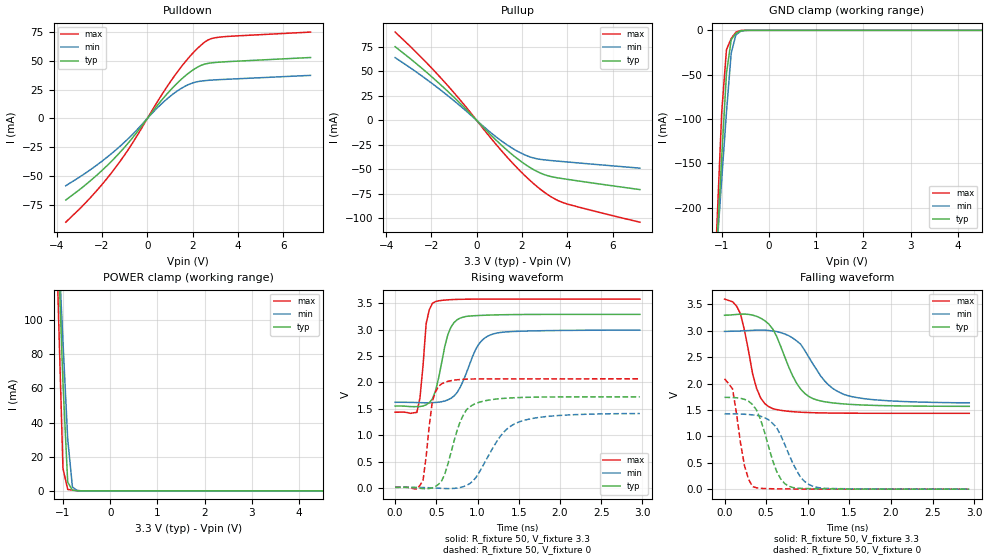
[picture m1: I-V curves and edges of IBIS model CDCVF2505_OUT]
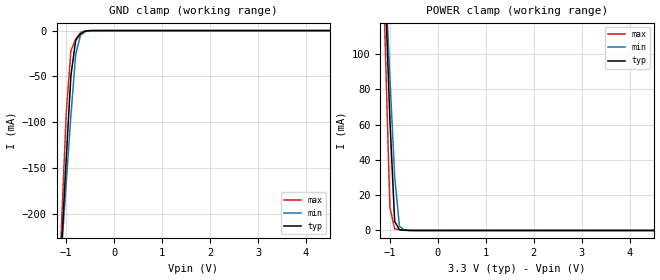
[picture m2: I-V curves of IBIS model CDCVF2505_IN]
|   TEXAS INSTRUMENTS INCORPORATED
|   CLOCK DISTRIBUTION CIRCUITS
|   IBIS Model of CDCVF2505
|   3.3-V High Performance PLL Clock Buffer
|   8-pin (PW(R), D(R)) Package
[IBIS Ver]   3.2
[File Name]   vf2505_2.ibs
[File Rev]   0.9
[Date]   Sept 6th 2005
[Source]   File originated at Texas Instruments, Inc.
[Notes]   The following is an IBIS list for the CDCVF2310.
|   - All test data contained in this file are derived from
|   hspice(tm) simulations.
|   - File created by HPA-Product Engineering.
|   01: model based on VF2310 simulation data. Tr seems to be about
|   200ps too fast compared to device characterization data.
|   0.8: Model correlated finally with updated package parasitics
|   to real silicon measurements.
|   0.9: Switched the definition of CLK_OUT pin - uses the same output model as the outputs 1Y0...1Y3.
|   But this pin is internally connected to "FBIN". C_comp therefore is different. In order to separately
|   add model data for this pin, also Hspice simulations would be needed. This pin normally is not used
|   in application to drive system loads. It acts mainly for phase adjustments to get the correct phase
|   between CLK and output buffers. But this effect is not modeled in IBIS.
|   If a customer needs this pin to drive system load, one may consider to increase C_comp by 2.4pF.
[Disclaimer] Property of Texas Instruments Incorporated.  Unauthorized
   reproduction and/or distribution is strictly prohibited.
   This product is protected under copyright law.
   Created 2004, (C) Copyright 2004, Texas Instruments Inc.,
   All Rights Reserved
   UNLESS THERE IS A SIGNED, WRITTEN AGREEMENT TO THE
   CONTRARY, TEXAS INSTRUMENTS ("TI") IS PROVIDING THE IBIS
   MODELS "AS IS" AND WITHOUT ANY WARRANTY, EXPRESSED OR
   IMPLIED.  TI assumes no liability for:
   1) the accuracy of the IBIS models provided to your
   company;
   2) the proper functioning of these IBIS models in your
   design or for any resulting applications; or
   3) infringement of patents, copyrights or intellectual
   property rights resulting from your use of these IBIS
   models.
   TI provides IBIS Models as a service to our customers.
   You and your company shall not distribute, sell or give
   these models to anyone else without prior written
   permission from TI.
   TI reserves the right to make changes to our products or
   to discontinue any semiconductor product or service
   without notice, and advises our customers to obtain the
   latest version of relevant information to verify, before
   placing orders, that the information being relied on is
   current.
   Please be aware that your receipt and use of the IBIS
   information provided shall serve as acceptance of these
   terms and conditions.  If you do not accept these terms,
   you should return or destroy the IBIS models and any
   other accompanying information immediately.
|   Model CDCVF2505PW(R)
[Component]   CDCVF2505PW   | (High_Performance_Clock_Buffer)
[Manufacturer]  Texas Instruments, Inc.
[Package]
|   typ   min   max
R_pkg   0.097ohm   0.067ohm   0.115ohm
L_pkg   3.349nH   2.836nH   3.571nH
C_pkg   0.308pF   0.263pF   0.371pF
[Pin]   signal_name   model_name   R_pin   L_pin   C_pin
  1   CLKIN   CDCVF2505_IN   0.099Ohm   3.541nH   0.343pF
  2   1Y1   CDCVF2505_OUT   0.104Ohm   3.297nH   0.263pF
  3   1Y0   CDCVF2505_OUT   0.109Ohm   3.365nH   0.272pF
  4   GND   GND   0.081Ohm   3.275nH   0.371pF
  5   1Y2   CDCVF2505_OUT   0.098Ohm   3.479nH   0.340pF
  6   VDD   POWER   0.067Ohm   2.836nH   0.319pF
  7   1Y3   CDCVF2505_OUT   0.115Ohm   3.430nH   0.275pF
| 8   CLKOUT   CDCVF2505_CLKOUT   0.102Ohm   3.571nH   0.284pF
|   Model CDCVF2505D(R)
[Component]   CDCVF2505D   | (High_Performance_Clock_Buffer)
[Manufacturer]  Texas Instruments, Inc.
[Package]
|   typ   min   max
R_pkg   0.087ohm   0.041ohm   0.113ohm
L_pkg   1.932nH   1.186nH   2.417nH
C_pkg   0.410pF   0.344pF   0.540pF
[Pin]   signal_name   model_name   R_pin   L_pin   C_pin
  1   CLKIN   CDCVF2505_IN   0.110Ohm   2.376nH   0.429pF
  2   1Y1   CDCVF2505_OUT   0.088Ohm   1.771nH   0.344pF
  3   1Y0   CDCVF2505_OUT   0.086Ohm   1.750nH   0.346pF
  4   GND   GND   0.060Ohm   1.756nH   0.540pF
  5   1Y2   CDCVF2505_OUT   0.111Ohm   2.400nH   0.429pF
  6   VDD   POWER   0.041Ohm   1.186nH   0.416pF
  7   1Y3   CDCVF2505_OUT   0.090Ohm   1.797nH   0.345pF
  8   CLKOUT   CDCVF2505_OUT   0.113Ohm   2.417nH   0.432pF
| Models and submodels in the file (2): CDCVF2505_OUT (3-state), CDCVF2505_IN (Input)
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|   Model CDCVF2505_OUT
[Model]   CDCVF2505_OUT
Model_type   3-state
Polarity   Non-Inverting
Enable   Active-High
Vmeas = 1.65V   |Vref for timing measurements.
Cref = 25pF   |load capacitance for timing spec.
Rref = 500   |500 Ohm to GND.
Vref = 0   |Timing specification test load voltage, GND
| variable   typ   min   max
C_comp   2.5pF   NA   NA
[Model Spec]
|  subparameter   typ   min   max
Vmeas   1.65V   1.5V   1.80V
[Temperature Range]   40   85   -40
[Voltage range]   3.3   3.0   3.6
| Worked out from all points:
|   slope of the pulldown table from 0 to 0.495 V, typ, clamps not added: 39.3 ohm
|   slope of the pullup table from 0 to 0.495 V, typ, clamps not added: 41.4 ohm
|   GND clamp passes 1 mA (typ) near -0.61 V on its own axis
|   POWER clamp passes 1 mA (typ) near -0.81 V on its own axis
|   rising waveform, R_fixture 50, V_fixture 3.3: 20-80 % time 151ps typ, 227ps min, 70.9ps max; typ from 1.55 V to 3.29 V
|   rising waveform, R_fixture 50, V_fixture 0: 20-80 % time 208ps typ, 349ps min, 92.9ps max; typ from 0.015 V to 1.73 V
|   falling waveform, R_fixture 50, V_fixture 3.3: 20-80 % time 299ps typ, 375ps min, 181ps max; typ from 3.29 V to 1.57 V
|   falling waveform, R_fixture 50, V_fixture 0: 20-80 % time 211ps typ, 257ps min, 125ps max; typ from 1.74 V to 0.001 V
|Process range|   nominal   weak   strong
[Pullup]
|   40C:3.3V:nominal   85C:3.0V:weak   -40C:3.6V:strong
|Voltage   I(typ)   I(min)   I(max)
-3.6V     75.26mA    64.11mA    90.19mA
-2.5V     54.79mA    46.69mA    65.63mA
-1.4V     32.29mA    27.52mA    38.67mA
-500mV    12.07mA    10.29mA    14.45mA
500mV     -12.07mA   -10.16mA   -14.59mA
1.2V      -27.57mA   -22.74mA   -33.79mA
1.7V      -37.39mA   -30.22mA   -46.45mA
2.1V      -44.29mA   -34.98mA   -55.81mA
2.8V      -53.66mA   -39.73mA   -70.14mA
3.4V      -57.95mA   -41.22mA   -79.6mA
3.9V      -59.82mA   -42.24mA   -84.63mA
7.2V      -70.62mA   -48.74mA   -103.9mA
[Pulldown]
|   40C:3.3V:nominal   85C:3.0V:weak   -40C:3.6V:strong
|   Voltage   I(typ)   I(min)   I(max)
-3.6V     -70.88mA   -58.48mA   -90.14mA
-2.4V     -52.25mA   -42.98mA   -66.38mA
-1.3V     -31.45mA   -25.82mA   -39.91mA
-600mV    -15.53mA   -12.8mA    -19.7mA
400mV     10.26mA    8.335mA    13.15mA
1.1V      26.26mA    20.67mA    34.21mA
1.8V      39.02mA    29.25mA    52.14mA
2.2V      44.39mA    31.86mA    60.58mA
2.5V      47mA       32.73mA    65.8mA
2.8V      48.16mA    33.24mA    69.16mA
3.3V      49.04mA    33.8mA     70.83mA
7.2V      52.9mA     37.39mA    74.99mA
[GND CLAMP]
|   40C:3.3V:nominal   85C:3.0V:weak   -40C:3.6V:strong
|   Voltage   I(typ)   I(min)   I(max)
-3.6V     -2.711A    -2.15A     -3.417A
-1.2V     -339.5mA   -320.2mA   -345.4mA
-1.1V     -240.7mA   -244mA     -217.5mA
-1V       -142.4mA   -167.9mA   -92.25mA
-900mV    -48.93mA   -92.6mA    -21.84mA
-800mV    -10.62mA   -25.94mA   -9.2mA
-700mV    -3.38mA    -5.012mA   -2.1mA
-600mV    -584.9uA   -1.132mA   -168.9uA
-400mV    -2.829uA   -16.92uA   -75.06nA
6.6V      158.6pA    496.2pA    154.8pA
[POWER CLAMP]
|   40C:3.3V:nominal   85C:3.0V:weak   -40C:3.6V:strong
|   Voltage   I(typ)   I(min)   I(max)
-3.6V     2.062A     1.625A     2.608A
-1.2V     216.4mA    205.4mA    208.3mA
-1.1V     139.5mA    146.2mA    108.3mA
-1V       63.07mA    87.18mA    13.12mA
-900mV    5.167mA    30.47mA    874.7uA
-800mV    396uA      2.327mA    462.6uA
-700mV    140.5uA    202.1uA    209.6uA
6.9V      -92.2pA    -171.3pA   -82.8pA
[ramp]
| variable   typ   min   max
|dV/dt_r   1.0433/2.3645E-10   0.8547/4.1361E-10   1.2533/1.1304E-10
dV/dt_r   1.0433/2.1208E-10   0.8547/3.5796E-10   1.2533/9.6403E-11
dV/dt_f   1.0483/3.0459E-10   0.8254/3.8579E-10   1.2981/1.8057E-10
R_load = 50ohms
[Rising Waveform]
R_fixture = 50
V_fixture = 3.3
V_fixture_min = 3.0
V_fixture_max = 3.6
|   40C:3.3V:nominal   85C:3.0V:weak  -40C:3.6V:strong
|   Time   V(typ)   V(min)   V(max)
0s        1.553V     1.624V     1.437V
263.2ps   1.542V     1.619V     1.432V
300.8ps   1.545V     1.617V     1.703V
376ps     1.576V     1.615V     3.111V
488.8ps   1.837V     1.621V     3.529V
639.2ps   2.902V     1.67V      3.563V
789.6ps   3.218V     1.908V     3.573V
977.6ps   3.264V     2.626V     3.576V
1.166ns   3.276V     2.905V     3.577V
2.97ns    3.289V     2.99V      3.578V
[Rising Waveform]
R_fixture = 50
V_fixture = 0
|   40C:3.3V:nominal   85C:3.0V:weak  -40C:3.6V:strong
|   Time   V(typ)   V(min)   V(max)
0s        15.2mV     13.3mV     15.5mV
263.2ps   3.5mV      14mV       -20.1mV
338.4ps   -9.6mV     11.2mV     146.5mV
451.2ps   4.9mV      4.7mV      1.641V
601.6ps   260.5mV    -7.9mV     2V
789.6ps   1.259V     11.1mV     2.055V
977.6ps   1.601V     194.6mV    2.066V
1.278ns   1.694V     985.6mV    2.068V
1.504ns   1.714V     1.252V     2.068V
2.97ns    1.727V     1.412V     2.068V
[Falling Waveform]
R_fixture = 50
V_fixture = 3.3
V_fixture_min = 3.0
V_fixture_max = 3.6
|   40C:3.3V:nominal   85C:3.0V:weak  -40C:3.6V:strong
|   Time   V(typ)   V(min)   V(max)
0s        3.293V     2.987V     3.6V
192.8ps   3.314V     2.996V     3.316V
385.6ps   3.273V     3.011V     1.907V
482ps     3.192V     3.011V     1.623V
578.4ps   3.036V     2.996V     1.526V
867.6ps   2.002V     2.807V     1.462V
1.06ns    1.717V     2.376V     1.448V
1.253ns   1.643V     1.97V      1.442V
1.494ns   1.607V     1.766V     1.439V
2.94ns    1.569V     1.637V     1.437V
[Falling Waveform]
R_fixture = 50
V_fixture = 0
|   40C:3.3V:nominal   85C:3.0V:weak   -40C:3.6V:strong
|   Time   V(typ)   V(min)   V(max)
0s        1.739V     1.425V     2.089V
96.4ps    1.735V     1.425V     1.898V
241ps     1.701V     1.419V     435.7mV
337.4ps   1.601V     1.406V     49.3mV
433.8ps   1.315V     1.381V     16.6mV
626.6ps   336.7mV    1.165V     6.6mV
771.2ps   56.5mV     665.3mV    4.1mV
915.8ps   15.8mV     219.7mV    2.7mV
1.109ns   8.1mV      35.5mV     1.7mV
2.94ns    600uV      900uV      400uV
|   Model CDCVF2505_IN
[Model]   CDCVF2505_IN
Model_type   Input
Polarity   Non-Inverting
Vinl = 0.99V
Vinh = 2.31V
| variable   typ   min   max
C_comp   3.8pF   NA   NA
[Model Spec]
|  subparameter   VCC=3.3V   VCC=3.0V   VCC=3.6V
Vinl   0.99V   0.9V   1.08V
Vinh   2.31V   2.1V   2.52V
[Temperature Range]   40   85   -40
[Voltage range]   3.3   3.0   3.6
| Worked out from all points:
|   GND clamp passes 1 mA (typ) near -0.61 V on its own axis
|   POWER clamp passes 1 mA (typ) near -0.81 V on its own axis
|Process range|   nominal   weak   strong
[GND CLAMP]
|   40C:3.3V:nominal   85C:3.0V:weak   -40C:3.6V:strong
|   Voltage   I(typ)   I(min)   I(max)
-3.6V     -2.711A    -2.15A     -3.417A
-1.2V     -339.5mA   -320.2mA   -345.4mA
-1.1V     -240.7mA   -244mA     -217.5mA
-1V       -142.4mA   -167.9mA   -92.25mA
-900mV    -48.93mA   -92.6mA    -21.84mA
-800mV    -10.62mA   -25.94mA   -9.2mA
-700mV    -3.38mA    -5.012mA   -2.1mA
-600mV    -584.9uA   -1.132mA   -168.9uA
-400mV    -2.829uA   -16.92uA   -75.06nA
6.6V      158.6pA    496.2pA    154.8pA
[POWER CLAMP]
|   40C:3.3V:nominal   85C:3.0V:weak   -40C:3.6V:strong
|   Voltage   I(typ)   I(min)   I(max)
-3.6V     2.062A     1.625A     2.608A
-1.2V     216.4mA    205.4mA    208.3mA
-1.1V     139.5mA    146.2mA    108.3mA
-1V       63.07mA    87.18mA    13.12mA
-900mV    5.167mA    30.47mA    874.7uA
-800mV    396uA      2.327mA    462.6uA
-700mV    140.5uA    202.1uA    209.6uA
6.9V      -92.2pA    -171.3pA   -82.8pA
